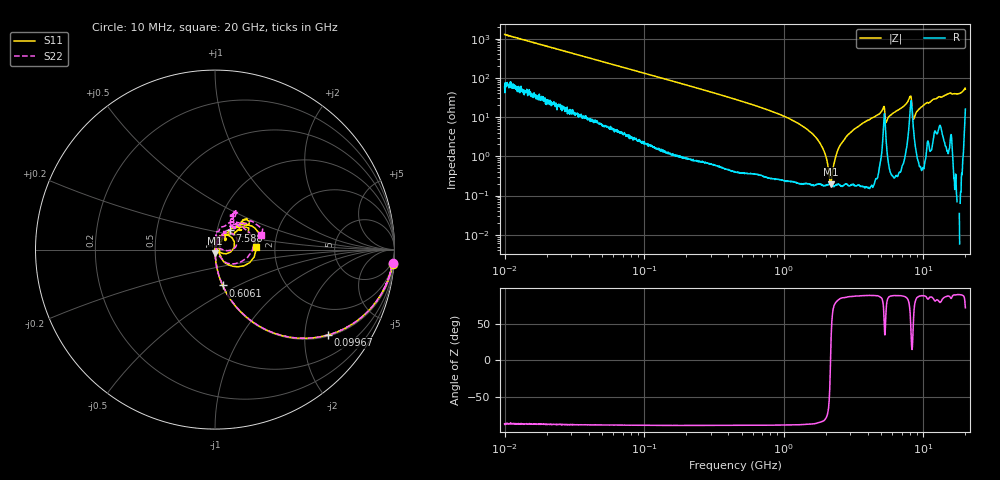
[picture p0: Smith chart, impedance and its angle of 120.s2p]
!Keysight Technologies,P5008B,MY61100088,A.16.20.02
!Date: Friday, August 30, 2024 13:32:43
!Correction: S11(C  2-Port  )
!S21(C  2-Port  )
!S12(C  2-Port  )
!S22(C  2-Port  )
!S2P File: Measurements: S11, S21, S12, S22:Log Frequency Sweep
# Hz S  MA  R 50
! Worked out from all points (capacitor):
!   1601 points, 10 MHz to 20 GHz, reference 50 ohm
!   read as one part in series: C = 12.5 pF near 10.39 MHz
!   lowest |Z| = 193 mohm at 2.165 GHz (marker M1)
!   series resonance near 2.162 GHz, so ESL is about 430 pH
!   S11 on the Smith chart (normalised r, x): 10 MHz: 2, -25; 99.67 MHz: 1.03, -2.62; 606.1 MHz: 1.00, -0.42; 7.588 GHz: 1.15, +0.25; 20 GHz: 1.59, +0.05
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1e7  0.9938 -4.5  0.07796 82.8  0.07799 82.9  0.9933 -4.5
3.555162e7  0.9571 -15.3  0.2628 73.0  0.2628 73.0  0.9569 -15.3
9.966934e7  0.7903 -37.0  0.6005 52.1  0.6004 52.1  0.7904 -37.0
1.263918e8  0.716 -43.6  0.6877 45.6  0.6874 45.6  0.7162 -43.6
4.472136e8  0.2768 -73.7  0.9569 15.6  0.9567 15.6  0.2768 -73.7
6.061166e8  0.2039 -78.1  0.9756 11.1  0.9753 11.1  0.2039 -77.9
1.589917e9  0.05272 -86.5  0.9967 1.4  0.9964 1.4  0.05294 -87.0
2.165104e9  0.0201 -85.0  0.998 -1.2  0.9979 -1.2  0.02047 -86.1
2.70674e9  0.00171 -138.1  0.9985 -3.1  0.9983 -3.1  0.005967 -27.4
3.211587e9  0.01719 91.5  0.9983 -4.7  0.9982 -4.8  0.01712 65.4
5.091486e9  0.08724 64.5  0.9773 -12.0  0.9771 -12.1  0.0926 65.9
5.493573e9  0.0139 51.7  0.9882 -8.7  0.988 -8.7  0.02632 30.5
5.652411e9  0.02955 77.4  0.9949 -9.8  0.9947 -9.9  0.036 60.1
7.588373e9  0.1355 52.1  0.9783 -18.2  0.978 -18.4  0.1287 75.5
8.148841e9  0.2292 0.4  0.7942 -17.6  0.794 -17.7  0.2192 9.0
8.750704e9  0.03128 -42.5  0.9845 -13.8  0.9844 -13.9  0.01886 -56.8
9.003717e9  0.0273 4.9  0.993 -15.4  0.9928 -15.6  0.01121 83.4
1.033363e10  0.07834 52.1  0.9927 -21.0  0.9924 -21.2  0.07837 69.6
1.273595e10  0.1687 40.6  0.9516 -26.6  0.9514 -26.8  0.1686 53.9
1.525565e10  0.2426 44.7  0.9654 -32.2  0.9652 -32.4  0.2392 61.5
1.827386e10  0.1607 48.5  0.9907 -39.4  0.9905 -39.7  0.1597 52.4
2e10  0.2295 3.9  0.8365 -43.6  0.8366 -43.9  0.2702 17.0
